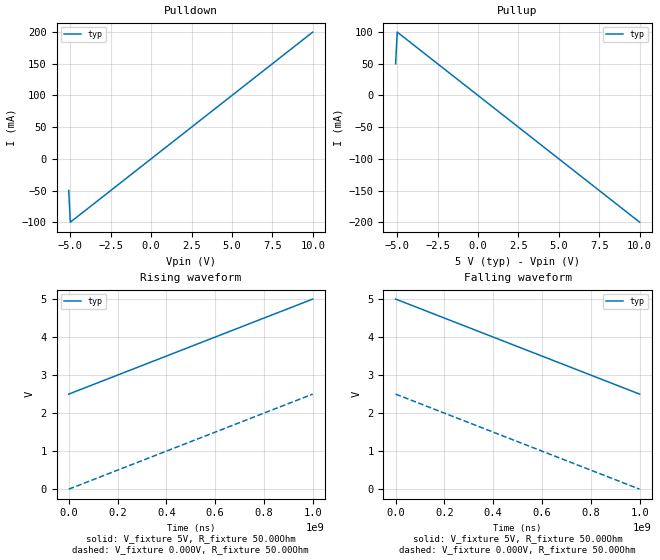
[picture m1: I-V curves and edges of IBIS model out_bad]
|********************* IBIS GOLDEN PARSER BUG REPORT FORM *********************
|INSTRUCTIONS
|To report a bug in the IBIS golden parser.  Please fill out the top part
|of the following form and send the complete form to ibischk-bug@vhdl.org.
|A list of reported bugs will be maintained on vhdl.org.
|PARSER VERSION NUMBER:
|   Found in IBISCHK3 V3.2.7
|PLATFORM (SPARC, HP700, PC, etc.):
|   Sun Ultra 10
|OS AND VERSION:
|   Unix Sun Solaris 5.
|REPORTED BY:
|   Bob Ross, Mentor Graphics
|DATE:
|   June 15, 2001
|DESCRIPTION OF BUG:
|   Non-Monotonic I-V Table Causes Waveform End Point Test to Fail
|INSERT IBIS FILE DEMONSTRATING THE BUG:
[IBIS Ver]   3.2
[File name]   bug57.ibs
[File rev]   0.1
[Date]   June 15, 2001
[Component]   BUG57
[Manufacturer]  Sample
[Package]
|   typ   min   max
R_pkg   0   NA NA
L_pkg   0   NA NA
C_pkg   0   NA NA
[Pin]  signal_name   model_name   R_pin   L_pin   C_pin
1  test   out_bad
| Models and submodels in the file (1): out_bad (Output)
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[Model]   out_bad
Model_type   Output
Vmeas = 2.5
Vref = 0
Cref = 5.00pF
C_comp   0   NA NA
[Voltage Range]  5.0 NA NA
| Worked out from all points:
|   slope of the pulldown table from 0 to 0.75 V, typ, clamps not added: 50 ohm
|   slope of the pullup table from 0 to 0.75 V, typ, clamps not added: 50 ohm
|   falling waveform, V_fixture 5V, R_fixture 50.00Ohm: 20-80 % time 600ms typ, NA min, NA max; typ from 5 V to 2.5 V
|   rising waveform, V_fixture 5V, R_fixture 50.00Ohm: 20-80 % time 600ms typ, NA min, NA max; typ from 2.5 V to 5 V
|   rising waveform, V_fixture 0.000V, R_fixture 50.00Ohm: 20-80 % time 600ms typ, NA min, NA max; typ from 0 V to 2.5 V
|   falling waveform, V_fixture 0.000V, R_fixture 50.00Ohm: 20-80 % time 600ms typ, NA min, NA max; typ from 2.5 V to 0 V
[Pulldown]
|*** Commenting this line out gives 0 errors and warnings
-5.1V     -50mA      NA         NA
-5V       -100mA     NA         NA
0V        0A         NA         NA
10V       200mA      NA         NA
[Pullup]
|*** And commenting this line out gives 0 errors and warnings
-5.1V     50mA       NA         NA
-5V       100mA      NA         NA
0V        0A         NA         NA
10V       -200mA     NA         NA
[Ramp]
dV/dt_r   1.5/.6n NA NA
dV/dt_f   1.5/.6n NA NA
[Falling Waveform]
V_fixture = 5V
R_fixture = 50.00Ohm
0s        5V         NA         NA
1s        2.5V       NA         NA
[Rising Waveform]
V_fixture = 5V
R_fixture = 50.00Ohm
0s        2.5V       NA         NA
1s        5V         NA         NA
[Rising Waveform]
V_fixture = 0.000V
R_fixture = 50.00Ohm
0s        0V         NA         NA
1s        2.5V       NA         NA
[Falling Waveform]
V_fixture = 0.000V
R_fixture = 50.00Ohm
0s        2.5V       NA         NA
1s        0V         NA         NA
